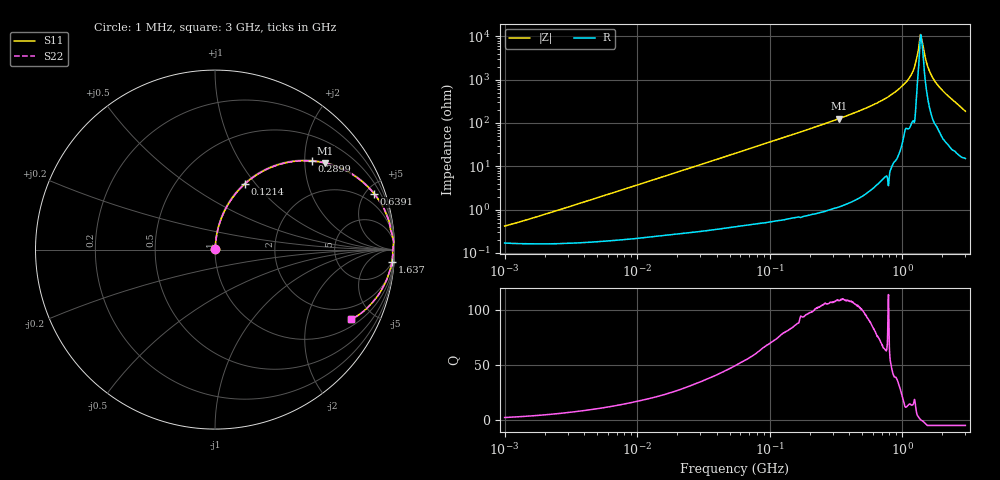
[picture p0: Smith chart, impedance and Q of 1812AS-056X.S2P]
!s-Parameter Generated by FASTRON Sdn. Bhd.
!FASTRON P/N : 1812AS-056X
!Keysight Technologies,E4991B,MY54100416,A.01.15
!Date created: Fri Oct 13 14:16:01 2023
!Version  : Rev00 Fri Oct 13 14:16:01 2023
!Data & Calibration Information:
!Freq	S11	S21	S12	S22
!PortZ  Port1:50+j0  Port2:50+j0
!When reading, reference impedance value at option line is always used.
! Remarks : This data is being provided solely for informational purposes.
# Hz S dB R 50
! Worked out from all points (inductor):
!   1601 points, 1 MHz to 3 GHz, reference 50 ohm
!   read as one part in series: L = 60.3 nH near 1.297 MHz
!   highest Q = 110 at 335.2 MHz (marker M1), where L = 60.2 nH
!   self-resonance near 1.381 GHz
!   S11 on the Smith chart (normalised r, x): 1 MHz: 1.00, +0.01; 121.4 MHz: 1.01, +0.88; 289.9 MHz: 1.02, +2.16; 639.1 MHz: 1.07, +5.70; 1.637 GHz: 5, -28; 3 GHz: 1.30, -3.72
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1000000  -47.63 65.8  -0.01 -0.2  -0.01 -0.2  -47.63 65.8
3804036  -36.88 82.3  -0.02 -0.8  -0.02 -0.8  -36.88 82.3
1.447069e7  -25.54 84.3  -0.03 -3.0  -0.03 -3.0  -25.54 84.3
5.477226e7  -14.27 77.7  -0.20 -11.2  -0.20 -11.2  -14.27 77.7
1.213667e8  -7.96 65.7  -0.81 -23.6  -0.81 -23.6  -7.96 65.7
2.083556e8  -4.39 52.3  -2.03 -37.1  -2.03 -37.1  -4.39 52.3
2.898922e8  -2.72 42.5  -3.40 -46.9  -3.40 -46.9  -2.72 42.5
3.351655e8  -2.14 38.1  -4.20 -51.4  -4.20 -51.4  -2.14 38.1
6.391491e8  -0.54 19.2  -9.64 -70.0  -9.64 -70.0  -0.54 19.2
7.925923e8  -0.27 13.6  -12.56 -75.8  -12.56 -75.8  -0.27 13.6
9.682285e8  -0.15 8.6  -16.46 -79.3  -16.46 -79.3  -0.15 8.6
1.159346e9  -0.08 4.6  -21.96 -81.4  -21.96 -81.4  -0.08 4.6
1.243477e9  -0.03 2.8  -26.23 -84.1  -26.23 -84.1  -0.03 2.8
1.287806e9  -0.05 1.8  -30.12 -78.7  -30.12 -78.7  -0.05 1.8
1.340405e9  -0.06 0.8  -35.93 -62.9  -35.93 -62.9  -0.06 0.8
1.381259e9  -0.08 0.1  -40.92 -6.3  -40.92 -6.3  -0.08 0.1
1.416254e9  -0.09 -0.4  -37.81 34.1  -37.81 34.1  -0.09 -0.4
1.526649e9  -0.09 -2.2  -28.00 74.7  -28.00 74.7  -0.09 -2.2
1.637435e9  -0.10 -4.0  -22.95 78.5  -22.95 78.5  -0.10 -4.0
1.791767e9  -0.16 -6.5  -18.86 77.5  -18.86 77.5  -0.16 -6.5
2.040726e9  -0.26 -10.3  -14.95 75.2  -14.95 75.2  -0.26 -10.3
3e9  -1.38 -27.1  -6.80 58.3  -6.80 58.3  -1.38 -27.1
